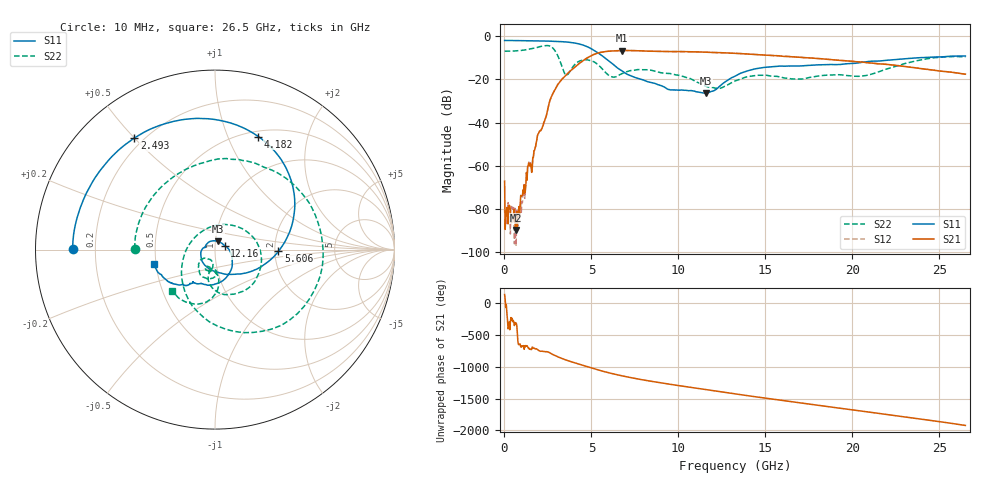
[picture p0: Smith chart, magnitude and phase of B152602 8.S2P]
!  2-Port S-parameters saved by WinCal
! VAR MeasName=S-Parameters (CALIBRATED_DATA) read from VNA (N5242A)
! VAR MeasDate=2016-1-5 16:26:39
! VAR NAME=B152602 8
! VAR FILENAME=B152602 8.S2P
! VAR DATE=2016-1-5 16:26:39
! VAR PHYS_PORTS=1,2
# Hz S DB R 50
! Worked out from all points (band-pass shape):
!   801 points, 10 MHz to 26.5 GHz, reference 50 ohm
!   highest |S21| = -6.66 dB at 6.765 GHz (marker M1); lowest = -89.7 dB at 639.1 MHz (marker M2)
!   |S21| within 3 dB of the highest: 4.851 GHz to 16.66 GHz (11.81 GHz wide, 110 % of centre); 16.6741 GHz to 16.70452 GHz (30.42 MHz wide, 0.182 % of centre)
!   lowest |S11| = -26.4 dB at 11.57 GHz (marker M3), VSWR 1.10, Z = 51.4 + j4.67 ohm
!   |S11| at or under -10 dB: 5.77 GHz to 23.83 GHz (18.06 GHz wide, 122 % of centre)
!   |S22| runs from -24.2 to -4.4 dB; largest |S21 - S12| = 0.003
!   S11 on the Smith chart (normalised r, x): 10 MHz: 0.12, +0.00; 2.493 GHz: 0.17, +0.50; 4.182 GHz: 0.56, +1.30; 5.606 GHz: 2.09, -0.05; 12.16 GHz: 1.11, +0.05; 26.5 GHz: 0.49, -0.09
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1e7  -2.01 179.8  -67.09 137.5  -80.54 -118.8  -6.98 179.4
1.755625e8  -2.01 176.3  -83.74 97.7  -81.79 62.6  -6.95 169.2
6.391375e8  -2.06 166.8  -89.67 36.3  -93.00 -55.8  -6.84 140.6
9.040375e8  -2.10 161.4  -77.76 78.9  -77.21 92.1  -6.67 123.9
1.73185e9  -2.20 144.0  -52.78 12.0  -52.99 10.0  -5.50 64.7
2.493438e9  -2.30 125.8  -33.73 -44.4  -33.76 -44.5  -4.37 -13.5
2.857675e9  -2.39 115.9  -25.44 -96.1  -25.44 -96.3  -6.20 -71.0
3.221912e9  -2.53 105.0  -20.73 -140.1  -20.75 -140.2  -12.16 -138.4
3.58615e9  -2.74 92.8  -17.66 -177.1  -17.68 -177.2  -18.06 115.5
4.182175e9  -3.42 69.0  -13.37 131.1  -13.39 131.1  -12.15 2.4
4.447075e9  -3.96 56.8  -11.79 108.9  -11.80 109.0  -11.22 -24.6
5.606012e9  -9.02 -1.6  -7.41 14.5  -7.41 14.6  -15.03 -102.0
6.76495e9  -16.13 -62.5  -6.66 -61.9  -6.67 -61.9  -17.32 -86.2
8.851038e9  -22.48 -176.9  -7.05 -166.0  -7.04 -166.1  -16.68 -126.6
1.156626e10  -26.36 70.2  -7.41 80.4  -7.42 80.4  -23.14 -135.8
1.216229e10  -24.70 21.8  -7.62 57.0  -7.64 57.0  -24.10 -119.7
1.3255e10  -18.52 -35.6  -7.96 14.1  -7.95 14.1  -20.78 -97.5
1.553976e10  -14.04 -96.1  -9.03 -72.4  -8.99 -72.7  -18.56 -116.9
1.769208e10  -13.40 -116.8  -10.16 -152.4  -10.13 -152.4  -18.92 -102.8
2.004306e10  -12.62 -126.6  -11.70 121.3  -11.69 121.3  -18.50 -102.4
2.209604e10  -11.08 -135.1  -13.19 46.0  -13.14 45.6  -14.93 -83.3
2.65e10  -9.19 -166.9  -17.61 -122.4  -17.63 -122.7  -9.63 -136.0
